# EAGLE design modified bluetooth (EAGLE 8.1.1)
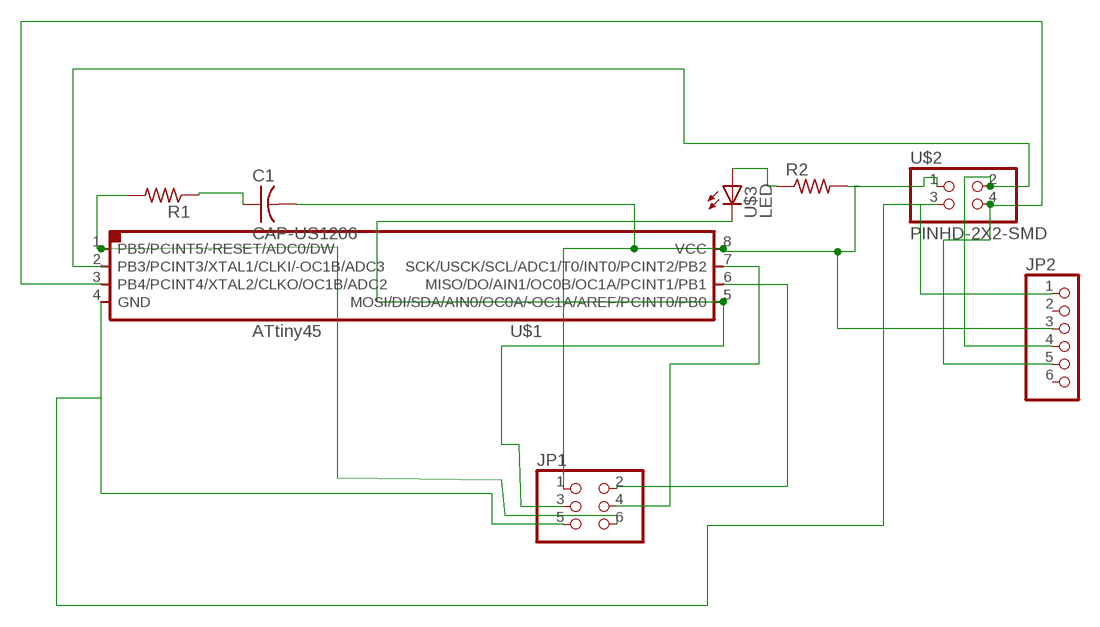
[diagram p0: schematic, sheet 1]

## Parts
C1  CAP-US1206  [C1206]
JP1  PINHD-2X3-SMD  [2X03SMD]
JP2  PINHD-1X6  [1X06]
R1  RES-US1206  [R1206]
R2  RES-US1206  [R1206]
U$1  ATTINY45SI  [SOIC8]
U$2  PINHD-2X2-SMD  [2X02SMD]
U$3  LED  [LED1206]

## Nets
N$1: C1.1 R1.1
N$2: JP1.6 R1.2 U$1.1(PB5/PCINT5/-RESET/ADC0/DW)
N$3: JP1.2 U$1.6(MISO/DO/AIN1/OC0B/OC1A/PCINT1/PB1)
N$4: JP1.3 U$1.5(MOSI/DI/SDA/AIN0/OC0A/-OC1A/AREF/PCINT0/PB0) U$3.2(C)
N$6: JP2.4 U$1.2(PB3/PCINT3/XTAL1/CLKI/-OC1B/ADC3) U$2.2
N$7: JP2.5 U$1.3(PB4/PCINT4/XTAL2/CLKO/OC1B/ADC2) U$2.4
N$8: R2.1 U$3.1(A)
N$9: R2.2 U$2.1
N$11: JP1.4 U$1.7(SCK/USCK/SCL/ADC1/T0/INT0/PCINT2/PB2)
N$13: C1.2 JP1.1 JP2.3 U$1.8(VCC)
N$15: JP1.5 JP2.1 U$1.4(GND) U$2.3
Unconnected: JP2.2 JP2.6

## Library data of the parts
C1 = fab:CAP-US
JP1 = fab:PINHD-2X3-SMD: PIN HEADER
JP2 = pinhead:PINHD-1X6: PIN HEADER
R1 R2 = fab:RES-US: Resistor (US Symbol)
U$1 = fab:ATTINY45
U$2 = fab:PINHD-2X2-SMD
U$3 = fab:LED: LED

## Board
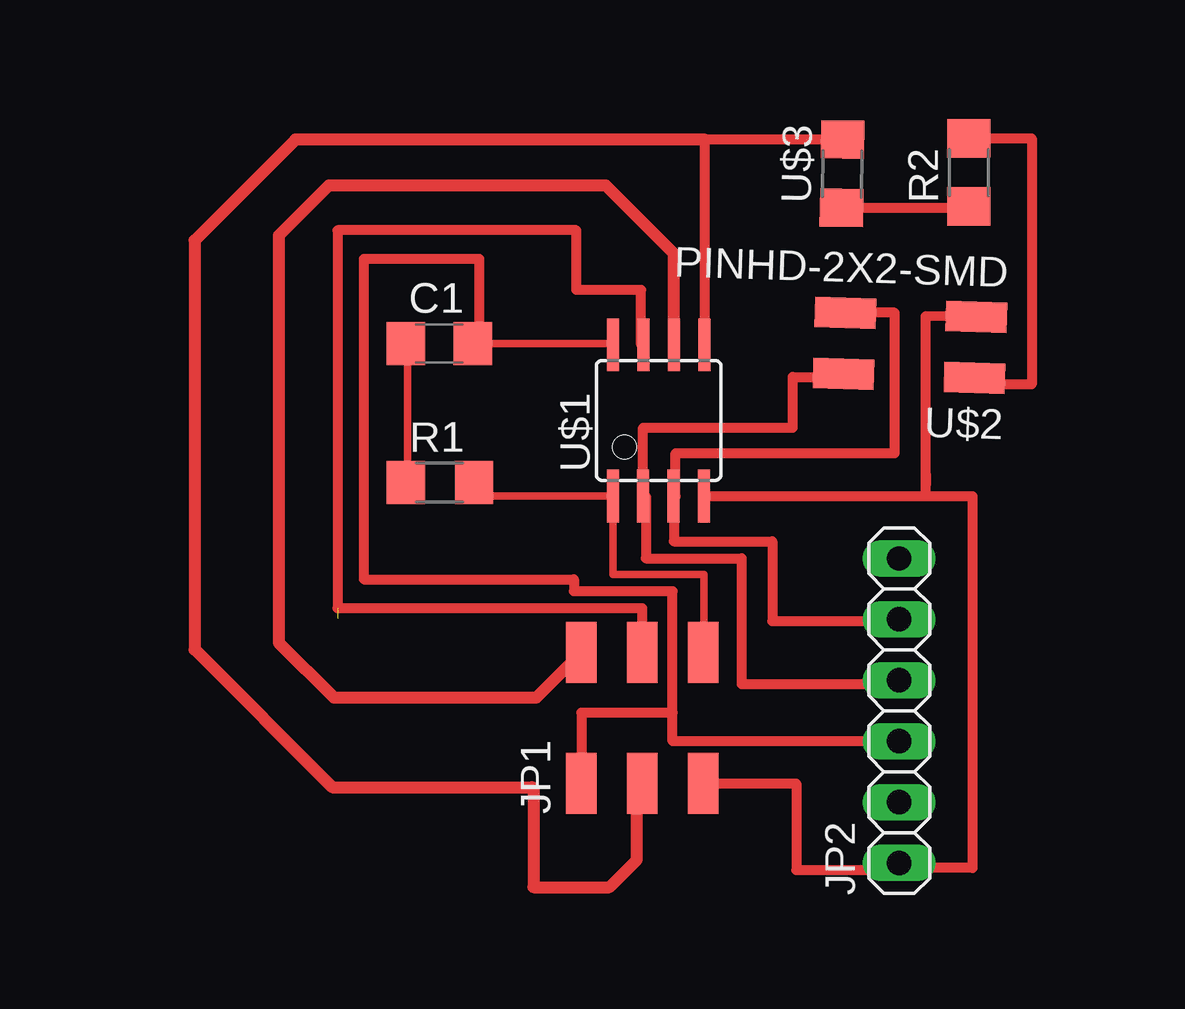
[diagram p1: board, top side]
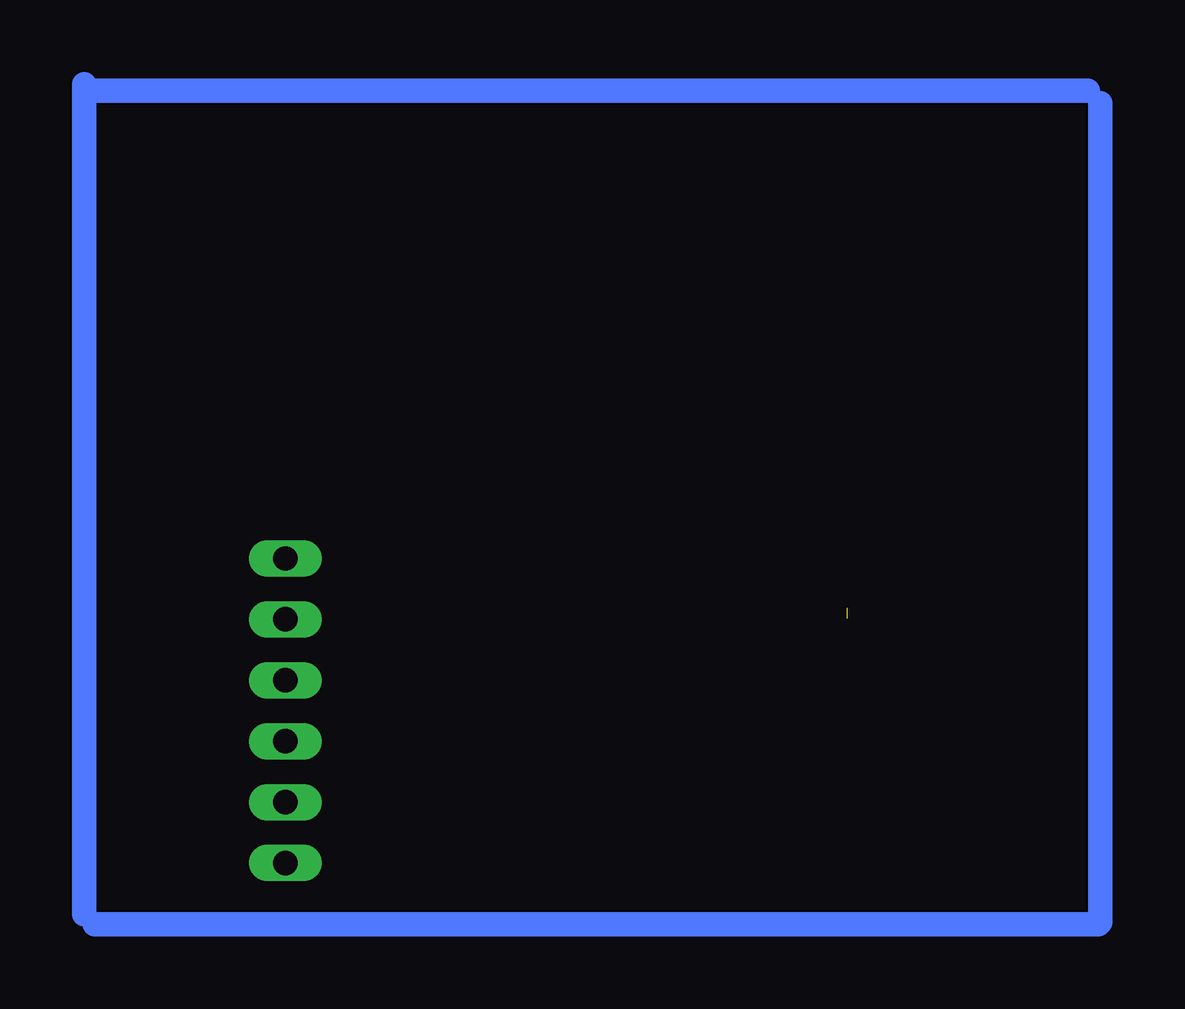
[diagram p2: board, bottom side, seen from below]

No outline drawn. Coordinates in mm, seen from the top.
Copper layers (1*16): Top 0.035mm / dielectric 1.5mm / Bottom 0.035mm
Design rules "default": minimum track width 10mil, minimum drill 24mil, track to track 8mil, track to pad 8mil, pad to pad 8mil, via to via 8mil, smd to smd 8mil, copper to edge 40mil, drill to drill 8mil, minimum pad ring 10mil, minimum via ring 8mil, stop-mask expansion 4mil, vias tented up to drill 0mil, thermal gap 10mil

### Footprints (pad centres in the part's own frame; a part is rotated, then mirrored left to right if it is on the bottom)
C1206 = smd 1.6 x 1.8: 1 -1.4,0; 2 1.4,0
2X03SMD = smd 2.54 x 1.27: 1 -2.54,2.54; 2 2.92,2.54; 3 -2.54,0; 4 2.92,0; 5 -2.54,-2.54; 6 2.92,-2.54
1X06 = drill 1.016 long: 1 -6.35,0; 2 -3.81,0; 3 -1.27,0; 4 1.27,0; 5 3.81,0; 6 6.35,0
R1206 = smd 1.6 x 1.803: 1 -1.422,0; 2 1.422,0
SOIC8 = smd 0.5 x 2.2: 1 -1.905,-3.154; 2 -0.645,-3.154; 3 0.625,-3.154; 4 1.895,-3.154; 5 1.905,3.154; 6 0.635,3.154; 7 -0.635,3.154; 8 -1.905,3.154
2X02SMD = smd 2.54 x 1.27: 1 -2.54,1.27; 2 2.92,1.27; 3 -2.54,-1.27; 4 2.92,-1.27
LED1206 = smd 1.6 x 1.803: 1 -1.422,0; 2 1.422,0

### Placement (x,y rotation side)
C1  26.42,23.52 0 top
JP1  34.87,7.72 90 top
JP2  45.59,8.22 90 top
R1  26.44,17.73 0 top
R2  48.49,30.66 90 top
U$1  35.56,20.32 0 top
U$2  46.23,23.44 178.2 top
U$3  43.21,30.61 89 top

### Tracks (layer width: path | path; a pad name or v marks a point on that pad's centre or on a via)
N$1
  Top 0.305: C1.1 25.09,23.52 25.09,17.09 25.02,17.09 R1.1
N$2
  Top 0.305: JP1.6 37.44,10.64 37.44,13.89 33.66,13.89 U$1.1 27.86,17.17 R1.2
N$3
  Top 0.305: 36.3,23.47 U$1.6 | JP1.2 32.33,9.7
  Top 0.508: U$1.6 36.2,27.28 33.35,30.12 21.81,30.12 19.73,28.03 19.73,11.06 22.02,8.77 30.46,8.77 JP1.2
N$4
  Top 0.305: JP1.3 35.08,5.18
  Top 0.406: U$3.2 37.47,32.03 U$1.5 | JP1.3 35.07,5.18
  Top 0.508: 37.47,32.03 20.43,32.03 16.21,27.82 16.21,10.77 21.95,5.03 30.27,5.03 30.34,4.96 30.34,0.86 33.5,0.86 34.65,2.01 34.65,4.96 JP1.3
N$5
  Bottom 0.508: 53.71,34.07 53.97,34.33 | 53.97,-0.26 53.54,-0.69 | 11.71,-0.69 11.62,-0.6 | 11.62,33.55 12.31,34.24
  Bottom 1.016: 12.14,34.07 53.71,34.07 | 53.97,34.33 53.97,-0.26 | 53.54,-0.69 11.71,-0.69 | 11.62,-0.6 11.62,33.55
N$6
  Top 0.305: 34.85,17.17 U$1.2
  Top 0.406: U$2.2 43.27,22.13 41.15,22.13 41.15,20.02 34.91,20.02 U$1.2 35.02,17.17 35.02,14.57 39.02,14.57 39.02,9.33 45.59,9.33 JP2.4
N$7
  Top 0.406: U$2.4 45.4,24.81 45.4,18.96 36.27,18.96 36.27,17.17 U$1.3 36.19,15.28 40.3,15.28 40.3,11.96 45.59,11.96 JP2.5
N$8
  Top 0.305: 43.18,29.24 U$3.1
  Top 0.406: U$3.1 48.49,29.18 R2.1
N$9
  Top 0.305: U$2.1 48.73,21.72
  Top 0.406: R2.2 51.1,32.08 51.1,21.82 48.73,21.82 U$2.1
N$11  (1 unrouted)
  Top 0.305: JP1.4 34.72,10.64
  Top 0.406: U$1.7 34.82,23.47 34.82,25.76 32.13,25.76 32.13,28.25 22.17,28.25 22.17,12.5 34.87,12.5 JP1.4
N$13
  Top 0.305: 33.63,23.47 U$1.8 33.66,23.52 C1.2 | JP1.1 32.56,5.18
  Top 0.406: C1.2 28.09,23.52 28.09,27.05 23.27,27.05 23.27,13.69 32.03,13.69 32.03,13.21 36.14,13.21 36.14,8.13 | 36.14,8.13 32.33,8.13 JP1.1 | 36.14,8.13 36.14,6.95 JP2.3
N$15
  Top 0.305: 37.41,5.08 JP1.5
  Top 0.406: 37.41,4.95 JP1.5 41.29,5.18 41.29,1.58 45.59,1.58 JP2.1 45.59,1.66 48.64,1.66 48.64,17.17 46.69,17.17 | U$2.3 46.69,24.66 46.69,18.11 | 46.69,18.11 46.69,17.61 | U$1.4 46.69,17.17 | 46.69,17.17 46.69,18.11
